(* Logix 5000 AddOnInstructionDefinition export YAI_Assy_155_119_EIP_Hz; software revision 21.03 *)

ADD_ON_INSTRUCTION YAI_Assy_155_119_EIP_Hz   (* revision 1.0, vendor Yaskawa America, Inc. *)
// YAI Assembly 155 and 119
// Help:
// This add-on instruction is for use with input assemblie 166 and output assemblies 116.
// Node_Input_Assy is defined as the node's input assembly integer array.
// Node_Output_Assy is defined as the node's output assembly integer array.
// Torque limit/reference, torque compensation and torque output variables are only available with A1000.
VAR_IN_OUT
   Node_Input_Assy : AB:ETHERNET_MODULE_INT_40Bytes:I:0; {required}   // Input assembly words
   Node_Output_Assy : AB:ETHERNET_MODULE_INT_18Bytes:O:0; {required}   // Output assembly words
END_VAR
VAR_INPUT
   RunFwd : BOOL; {visible}   // Forward run command
   RunRev : BOOL; {visible}   // Reverse run command
   MFI_3 : BOOL; {visible}   // Multi-function input 3
   MFI_4 : BOOL; {visible}   // Multi-function input 4
   MFI_5 : BOOL; {visible}   // Multi-function input 5
   MFI_6 : BOOL; {visible}   // Multi-function input 6
   MFI_7 : BOOL; {visible}   // Multi-function input 7
   MFI_8 : BOOL; {visible}   // Multi-function input 8
   External_Fault : BOOL;   // External fault command (EF0)
   FaultReset : BOOL; {visible}   // Fault reset command
   MFO_1 : BOOL; {visible}   // Multi-function output (M1-M2 for A/P1000, MA/MB/MC for V1000)
   MFO_2 : BOOL; {visible}   // Multi-function output (M3-M4 for A/P1000, P1 for V1000)
   MFO_3 : BOOL; {visible}   // Multi-function output (M5-M6 for A/P1000, P2 for V1000)
   Freq_Ref : REAL; {visible}   // Frequency reference command in Hz (xx.xx resolution)
   Digital_Output_Fault_Enable : BOOL;   // Bit to enable control of fault output relay over the network
END_VAR
VAR_OUTPUT
   Running : BOOL; {access Read Only, visible}   // Drive running forward status bit
   ZSP : BOOL; {access Read Only, visible}   // Drive zero speed status bit
   RunningRev : BOOL; {access Read Only, visible}   // Drive running reverse status bit
   Reset : BOOL; {access Read Only, visible}   // Drive reset command status bit
   At_Speed : BOOL; {access Read Only, visible}   // Drive at commanded speed status bit
   Ready : BOOL; {access Read Only, visible}   // Drive ready status bit
   Alarm : BOOL; {access Read Only, visible}   // Drive alarm status bit
   Faulted : BOOL; {access Read Only, visible}   // Drive faulted status bit
   OPE : BOOL; {access Read Only}   // OPE alarm/fault present
   UV : BOOL; {access Read Only}   // Drive in UV (undervoltage) state status bit
   NetCtrlStatus : BOOL; {access Read Only, visible}   // Drive network run source status bit (1 = source coming from network)
   MFO_1_Status : BOOL; {access Read Only, visible}   // Drive multi-function output 1 (M1-M2 for A/P1000, MA/MB/MC for V1000) status
   MFO_2_Status : BOOL; {access Read Only, visible}   // Drive multi-function output 1 (M3-M4 for A/P1000, P1 for V1000) status
   MFO_3_Status : BOOL; {access Read Only, visible}   // Drive multi-function output 1 (M5-M6 for A/P1000, P2 for V1000) status
   ZSV : BOOL; {access Read Only, visible}   // Drive zero servo completed status bit
   Motor_Speed : REAL; {access Read Only, visible}   // Motor speed in Hz (xx.xx resolution)
   Torque_Actual : REAL; {access Read Only, visible}   // Drive torque output in % (xxx.x resolution)
   PG1_Count : INT; {access Read Only}   // Encoder feedback count
   Freq_Cmd : REAL; {access Read Only, visible}   // Commanded frequency in Hz (xx.xx resolution)
   Output_Freq : REAL; {access Read Only, visible}   // Drive output frequency in Hz (xx.xx resolution)
   Output_Current : REAL; {access Read Only, visible}   // Drive output current in A (xxx.x resolution)
   Analog_Input_1_Level : REAL; {access Read Only}   // Analog input 1 level in % (xxx.x resolution)
   DC_Bus_Volt : INT; {access Read Only, visible}   // DC bus voltage in Vdc (xxx resolution)
   Analog_Input_3_Level : REAL; {access Read Only}   // Analog input 3 level in % (xxx.x resolution)
   Analog_Input_2_Level : REAL; {access Read Only}   // Analog input 2 level in % (xxx.x resolution)
   S1_Status : BOOL; {access Read Only}   // Digital input S1 status
   S2_Status : BOOL; {access Read Only}   // Digital input S2 status
   S3_Status : BOOL; {access Read Only}   // Digital input S3 status
   S4_Status : BOOL; {access Read Only}   // Digital input S4 status
   S5_Status : BOOL; {access Read Only}   // Digital input S5 status
   S6_Status : BOOL; {access Read Only}   // Digital input S6 status
   S7_Status : BOOL; {access Read Only}   // Digital input S7 status
   S8_Status : BOOL; {access Read Only}   // Digital input S8 status
   PG2_Count : INT;   // Encoder 2 feedback count
   UV_Alarm : BOOL; {access Read Only}   // Undervoltage alarm
   OV_Alarm : BOOL; {access Read Only}   // Overvoltage alarm
   OH_Alarm : BOOL; {access Read Only}   // Overheat alarm
   OH2_Alarm : BOOL; {access Read Only}   // Drive overheat alarm
   OL3_Alarm : BOOL; {access Read Only}   // Overtorque detection 1 alarm
   OL4_Alarm : BOOL; {access Read Only}   // Overtorque detection 2 alarm
   EF_Alarm : BOOL; {access Read Only}   // Run command error alarm
   bb_Alarm : BOOL; {access Read Only}   // Baseblock alarm
   EF3_Alarm : BOOL; {access Read Only}   // External fault 3 alarm
   EF4_Alarm : BOOL; {access Read Only}   // External fault 4 alarm
   EF5_Alarm : BOOL; {access Read Only}   // External fault 5 alarm
   EF6_Alarm : BOOL; {access Read Only}   // External fault 6 alarm
   EF7_Alarm : BOOL; {access Read Only}   // External fault 7 alarm
   EF8_Alarm : BOOL; {access Read Only}   // External fault 8 alarm
   FAN_Alarm : BOOL; {access Read Only}   // Cooling fan error alarm
   OS_Alarm : BOOL; {access Read Only}   // Overspeed alarm
   DEV_Alarm : BOOL; {access Read Only}   // Speed deviation alarm
   PGO_Alarm : BOOL; {access Read Only}   // Encoder feedback open alarm
   OPR_Alarm : BOOL; {access Read Only}   // Operator removed alarm
   CE_Alarm : BOOL; {access Read Only}   // Serial communication error alarm
   BUS_Alarm : BOOL; {access Read Only}   // BUS alarm
   CALL_Alarm : BOOL; {access Read Only}   // Serial communication timeout alarm
   OL1_Alarm : BOOL; {access Read Only}   // Motor overload alarm
   OL2_Alarm : BOOL; {access Read Only}   // Drive overload alarm
   EF0_Alarm : BOOL; {access Read Only}   // External fault 0 alarm
   RUN_Alarm : BOOL; {access Read Only}   // Motor 2 run command issued while running alarm
   UL3_Alarm : BOOL; {access Read Only}   // Undertorque detecxtion 1 alarm
   UL4_Alarm : BOOL; {access Read Only}   // Undertorque detection 2 alarm
   SE_Alarm : BOOL; {access Read Only}   // Modbus test failure alarm
   OH3_Alarm : BOOL; {access Read Only}   // Motor overload alarm
   FBL_Alarm : BOOL; {access Read Only}   // PID feedback loss alarm
   FBH_Alarm : BOOL; {access Read Only}   // PID feedback loss alarm
   DNE_Alarm : BOOL; {access Read Only}   // Drive not enabled alarm
END_VAR
VAR_INPUT
   Custom_Out_1 : INT;
   Custom_Out_2 : INT;
   Custom_Out_3 : INT;
   Custom_Out_4 : INT;
   Custom_Out_5 : INT;
   Custom_Out_6 : INT;
   Custom_Out_7 : INT;
END_VAR
VAR
   FRef_Convert : DINT;
   FOut_Convert : REAL;
   FOut_Temp : REAL;
   TRef_Convert : INT;
   TComp_Convert : INT;
   TOut_Convert : REAL;
   TOut_Temp : REAL;
   IOut_Temp : REAL;
   IOut_Convert : REAL;
   AO1_Convert : INT;
   AO2_Convert : INT;
   Motor_Speed_Temp : REAL;
   Motor_Speed_Convert : REAL;
   Freq_Cmd_Temp : REAL;
   Freq_Cmd_Convert : REAL;
   AI1_Temp : REAL;
   AI1_Convert : REAL;
   AI2_Temp : REAL; {access None}
   AI2_Convert : REAL; {access None}
   AI3_Temp : REAL; {access None}
   AI3_Convert : REAL; {access None}
END_VAR

ROUTINE Logic   (* ladder *)
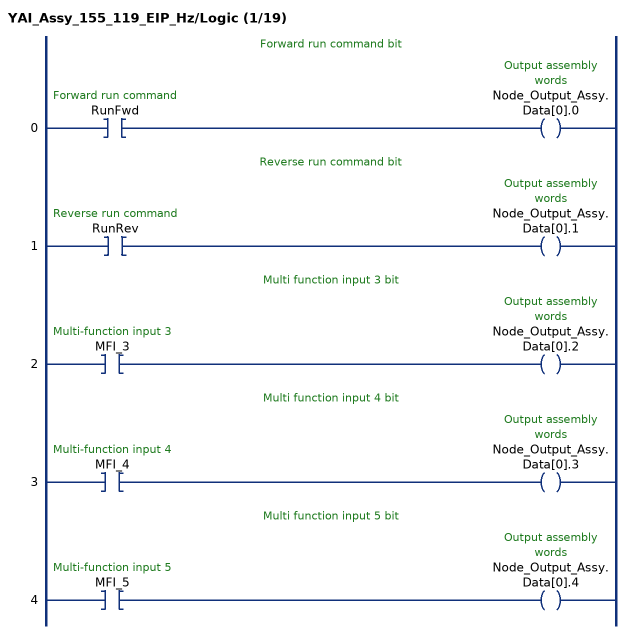
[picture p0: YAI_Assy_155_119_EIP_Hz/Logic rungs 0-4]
   // Forward run command bit
   0: XIC(RunFwd)OTE(Node_Output_Assy.Data[0].0);
   // Reverse run command bit
   1: XIC(RunRev)OTE(Node_Output_Assy.Data[0].1);
   // Multi function input 3 bit
   2: XIC(MFI_3)OTE(Node_Output_Assy.Data[0].2);
   // Multi function input 4 bit
   3: XIC(MFI_4)OTE(Node_Output_Assy.Data[0].3);
   // Multi function input 5 bit
   4: XIC(MFI_5)OTE(Node_Output_Assy.Data[0].4);
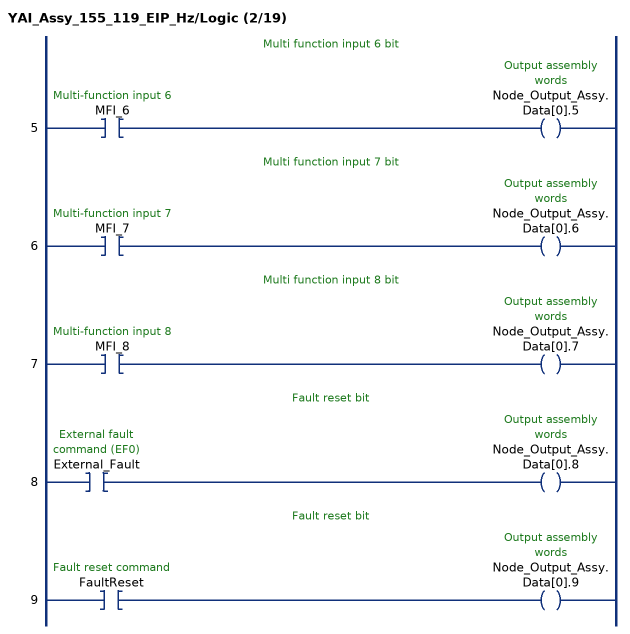
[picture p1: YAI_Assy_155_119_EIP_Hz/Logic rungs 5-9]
   // Multi function input 6 bit
   5: XIC(MFI_6)OTE(Node_Output_Assy.Data[0].5);
   // Multi function input 7 bit
   6: XIC(MFI_7)OTE(Node_Output_Assy.Data[0].6);
   // Multi function input 8 bit
   7: XIC(MFI_8)OTE(Node_Output_Assy.Data[0].7);
   // Fault reset bit
   8: XIC(External_Fault)OTE(Node_Output_Assy.Data[0].8);
   // Fault reset bit
   9: XIC(FaultReset)OTE(Node_Output_Assy.Data[0].9);
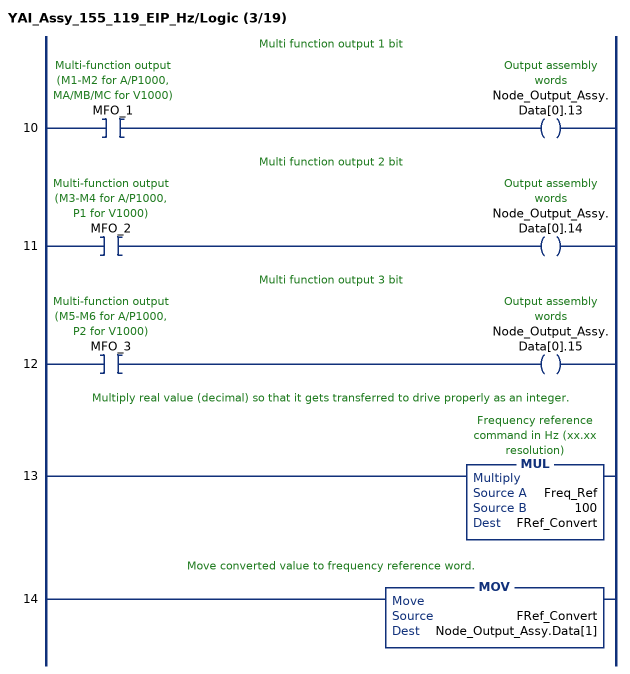
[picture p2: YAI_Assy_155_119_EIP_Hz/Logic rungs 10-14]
   // Multi function output 1 bit
   10: XIC(MFO_1)OTE(Node_Output_Assy.Data[0].13);
   // Multi function output 2 bit
   11: XIC(MFO_2)OTE(Node_Output_Assy.Data[0].14);
   // Multi function output 3 bit
   12: XIC(MFO_3)OTE(Node_Output_Assy.Data[0].15);
   // Multiply real value (decimal) so that it gets transferred to drive properly as an integer.
   13: MUL(Freq_Ref,100,FRef_Convert);
   // Move converted value to frequency reference word.
   14: MOV(FRef_Convert,Node_Output_Assy.Data[1]);
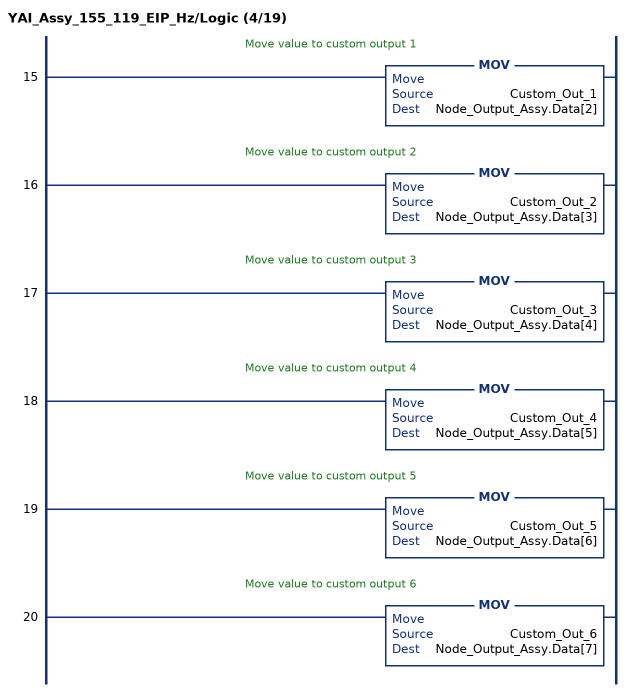
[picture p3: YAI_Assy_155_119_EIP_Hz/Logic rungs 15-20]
   // Move value to custom output 1
   15: MOV(Custom_Out_1,Node_Output_Assy.Data[2]);
   // Move value to custom output 2
   16: MOV(Custom_Out_2,Node_Output_Assy.Data[3]);
   // Move value to custom output 3
   17: MOV(Custom_Out_3,Node_Output_Assy.Data[4]);
   // Move value to custom output 4
   18: MOV(Custom_Out_4,Node_Output_Assy.Data[5]);
   // Move value to custom output 5
   19: MOV(Custom_Out_5,Node_Output_Assy.Data[6]);
   // Move value to custom output 6
   20: MOV(Custom_Out_6,Node_Output_Assy.Data[7]);
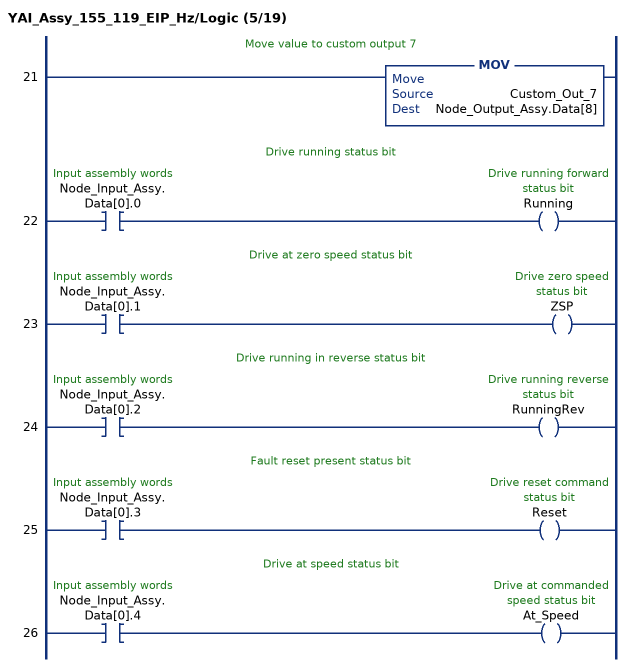
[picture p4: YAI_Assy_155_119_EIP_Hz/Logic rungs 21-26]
   // Move value to custom output 7
   21: MOV(Custom_Out_7,Node_Output_Assy.Data[8]);
   // Drive running status bit
   22: XIC(Node_Input_Assy.Data[0].0)OTE(Running);
   // Drive at zero speed status bit
   23: XIC(Node_Input_Assy.Data[0].1)OTE(ZSP);
   // Drive running in reverse status bit
   24: XIC(Node_Input_Assy.Data[0].2)OTE(RunningRev);
   // Fault reset present status bit
   25: XIC(Node_Input_Assy.Data[0].3)OTE(Reset);
   // Drive at speed status bit
   26: XIC(Node_Input_Assy.Data[0].4)OTE(At_Speed);
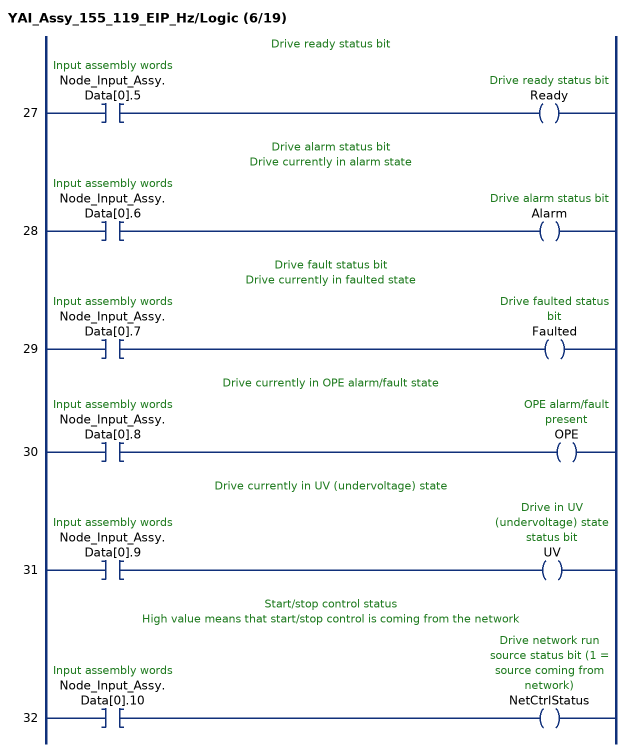
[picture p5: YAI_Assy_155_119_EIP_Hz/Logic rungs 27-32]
   // Drive ready status bit
   27: XIC(Node_Input_Assy.Data[0].5)OTE(Ready);
   // Drive alarm status bit
   // Drive currently in alarm state
   28: XIC(Node_Input_Assy.Data[0].6)OTE(Alarm);
   // Drive fault status bit
   // Drive currently in faulted state
   29: XIC(Node_Input_Assy.Data[0].7)OTE(Faulted);
   // Drive currently in OPE alarm/fault state
   30: XIC(Node_Input_Assy.Data[0].8)OTE(OPE);
   // Drive currently in UV (undervoltage) state
   31: XIC(Node_Input_Assy.Data[0].9)OTE(UV);
   // Start/stop control status
   // High value means that start/stop control is coming from the network
   32: XIC(Node_Input_Assy.Data[0].10)OTE(NetCtrlStatus);
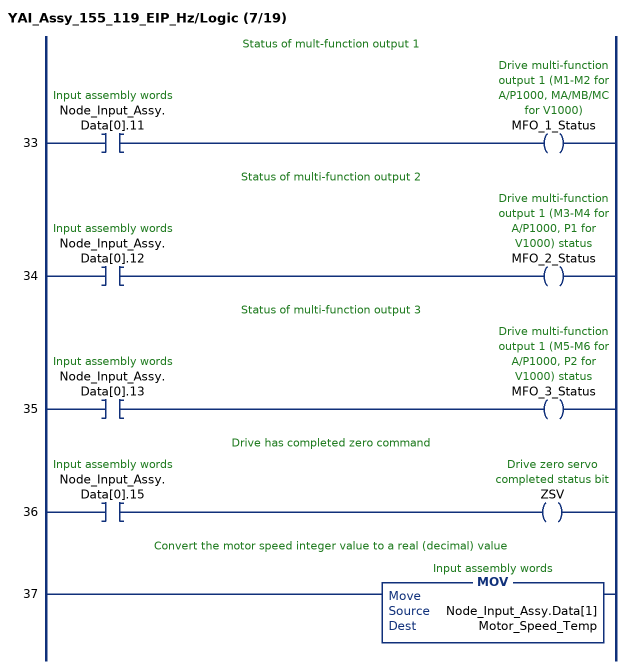
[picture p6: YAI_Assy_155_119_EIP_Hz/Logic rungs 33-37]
   // Status of mult-function output 1
   33: XIC(Node_Input_Assy.Data[0].11)OTE(MFO_1_Status);
   // Status of multi-function output 2
   34: XIC(Node_Input_Assy.Data[0].12)OTE(MFO_2_Status);
   // Status of multi-function output 3
   35: XIC(Node_Input_Assy.Data[0].13)OTE(MFO_3_Status);
   // Drive has completed zero command
   36: XIC(Node_Input_Assy.Data[0].15)OTE(ZSV);
   // Convert the motor speed integer value to a real (decimal) value
   37: MOV(Node_Input_Assy.Data[1],Motor_Speed_Temp);
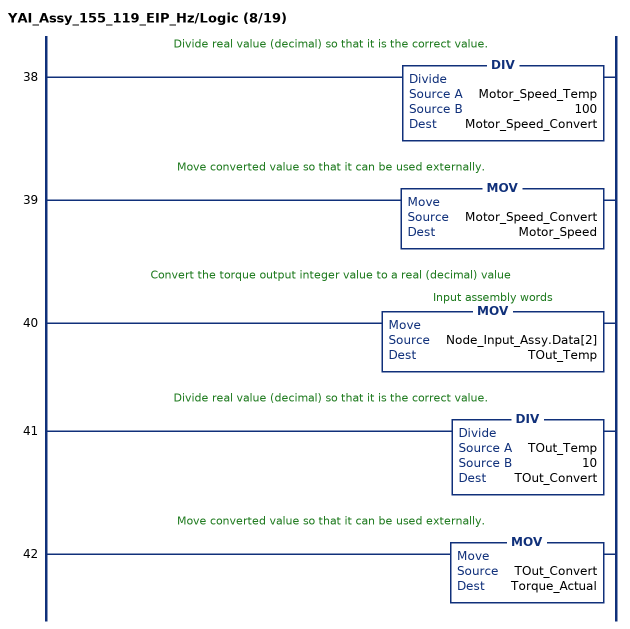
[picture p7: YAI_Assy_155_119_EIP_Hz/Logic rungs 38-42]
   // Divide real value (decimal) so that it is the correct value.
   38: DIV(Motor_Speed_Temp,100,Motor_Speed_Convert);
   // Move converted value so that it can be used externally.
   39: MOV(Motor_Speed_Convert,Motor_Speed);
   // Convert the torque output integer value to a real (decimal) value
   40: MOV(Node_Input_Assy.Data[2],TOut_Temp);
   // Divide real value (decimal) so that it is the correct value.
   41: DIV(TOut_Temp,10,TOut_Convert);
   // Move converted value so that it can be used externally.
   42: MOV(TOut_Convert,Torque_Actual);
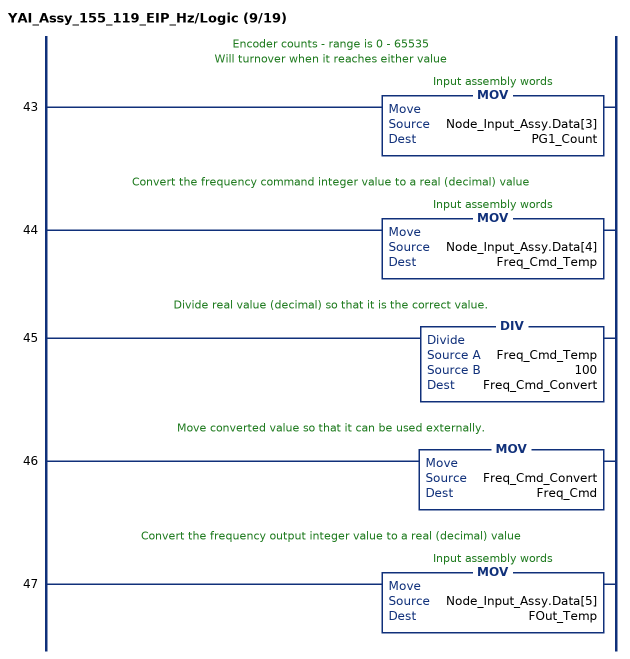
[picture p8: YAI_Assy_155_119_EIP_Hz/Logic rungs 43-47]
   // Encoder counts - range is 0 - 65535
   // Will turnover when it reaches either value
   43: MOV(Node_Input_Assy.Data[3],PG1_Count);
   // Convert the frequency command integer value to a real (decimal) value
   44: MOV(Node_Input_Assy.Data[4],Freq_Cmd_Temp);
   // Divide real value (decimal) so that it is the correct value.
   45: DIV(Freq_Cmd_Temp,100,Freq_Cmd_Convert);
   // Move converted value so that it can be used externally.
   46: MOV(Freq_Cmd_Convert,Freq_Cmd);
   // Convert the frequency output integer value to a real (decimal) value
   47: MOV(Node_Input_Assy.Data[5],FOut_Temp);
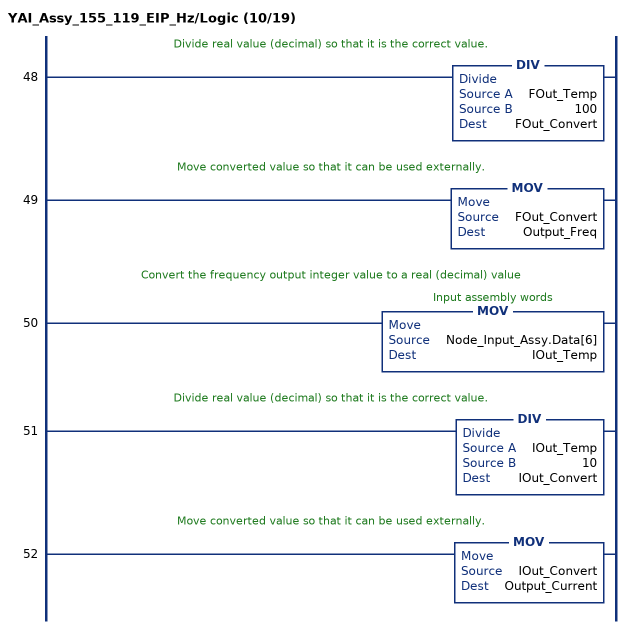
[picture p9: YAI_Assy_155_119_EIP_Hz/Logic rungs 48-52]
   // Divide real value (decimal) so that it is the correct value.
   48: DIV(FOut_Temp,100,FOut_Convert);
   // Move converted value so that it can be used externally.
   49: MOV(FOut_Convert,Output_Freq);
   // Convert the frequency output integer value to a real (decimal) value
   50: MOV(Node_Input_Assy.Data[6],IOut_Temp);
   // Divide real value (decimal) so that it is the correct value.
   51: DIV(IOut_Temp,10,IOut_Convert);
   // Move converted value so that it can be used externally.
   52: MOV(IOut_Convert,Output_Current);
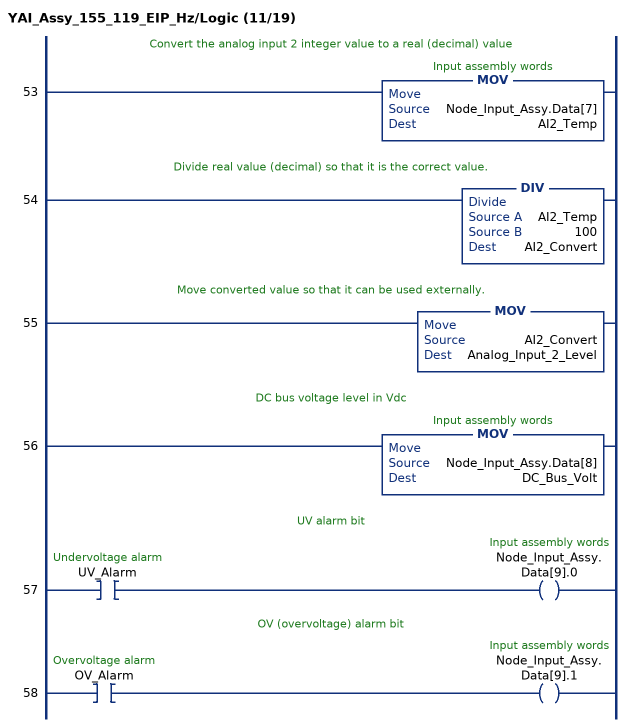
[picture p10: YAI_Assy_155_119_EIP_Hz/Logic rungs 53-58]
   // Convert the analog input 2 integer value to a real (decimal) value
   53: MOV(Node_Input_Assy.Data[7],AI2_Temp);
   // Divide real value (decimal) so that it is the correct value.
   54: DIV(AI2_Temp,100,AI2_Convert);
   // Move converted value so that it can be used externally.
   55: MOV(AI2_Convert,Analog_Input_2_Level);
   // DC bus voltage level in Vdc
   56: MOV(Node_Input_Assy.Data[8],DC_Bus_Volt);
   // UV alarm bit
   57: XIC(UV_Alarm)OTE(Node_Input_Assy.Data[9].0);
   // OV (overvoltage) alarm bit
   58: XIC(OV_Alarm)OTE(Node_Input_Assy.Data[9].1);
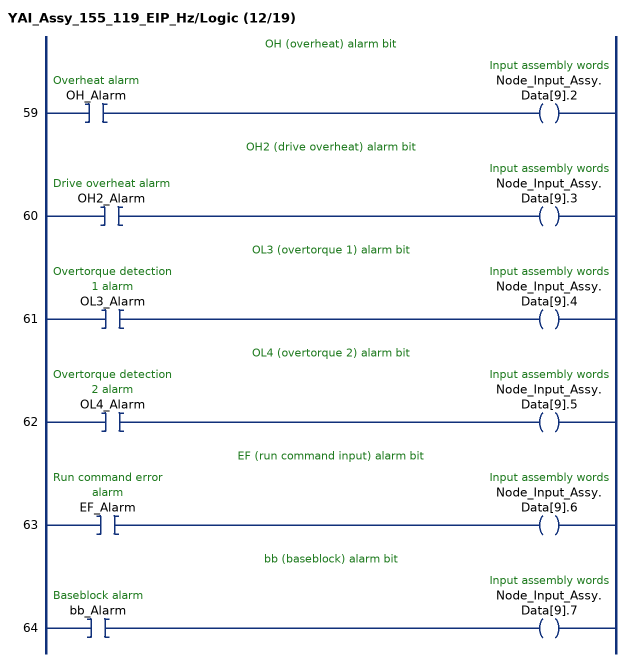
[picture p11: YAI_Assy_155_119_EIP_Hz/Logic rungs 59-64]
   // OH (overheat) alarm bit
   59: XIC(OH_Alarm)OTE(Node_Input_Assy.Data[9].2);
   // OH2 (drive overheat) alarm bit
   60: XIC(OH2_Alarm)OTE(Node_Input_Assy.Data[9].3);
   // OL3 (overtorque 1) alarm bit
   61: XIC(OL3_Alarm)OTE(Node_Input_Assy.Data[9].4);
   // OL4 (overtorque 2) alarm bit
   62: XIC(OL4_Alarm)OTE(Node_Input_Assy.Data[9].5);
   // EF (run command input) alarm bit
   63: XIC(EF_Alarm)OTE(Node_Input_Assy.Data[9].6);
   // bb (baseblock) alarm bit
   64: XIC(bb_Alarm)OTE(Node_Input_Assy.Data[9].7);
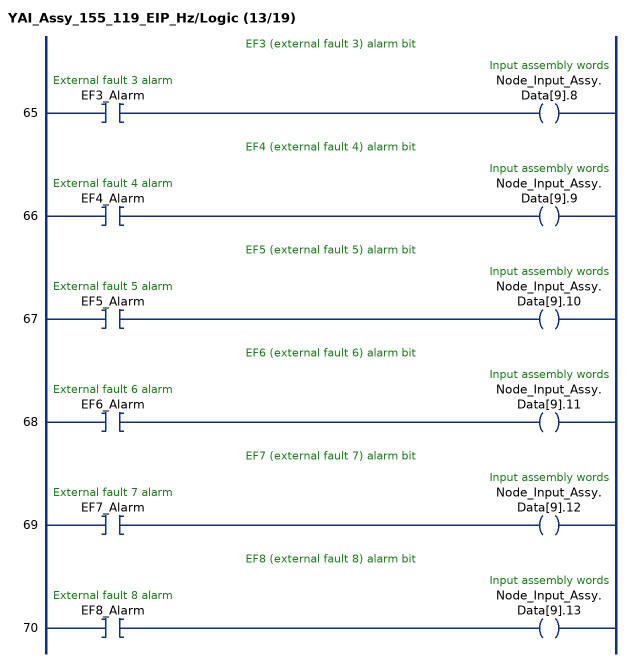
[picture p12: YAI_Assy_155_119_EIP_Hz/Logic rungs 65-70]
   // EF3 (external fault 3) alarm bit
   65: XIC(EF3_Alarm)OTE(Node_Input_Assy.Data[9].8);
   // EF4 (external fault 4) alarm bit
   66: XIC(EF4_Alarm)OTE(Node_Input_Assy.Data[9].9);
   // EF5 (external fault 5) alarm bit
   67: XIC(EF5_Alarm)OTE(Node_Input_Assy.Data[9].10);
   // EF6 (external fault 6) alarm bit
   68: XIC(EF6_Alarm)OTE(Node_Input_Assy.Data[9].11);
   // EF7 (external fault 7) alarm bit
   69: XIC(EF7_Alarm)OTE(Node_Input_Assy.Data[9].12);
   // EF8 (external fault 8) alarm bit
   70: XIC(EF8_Alarm)OTE(Node_Input_Assy.Data[9].13);
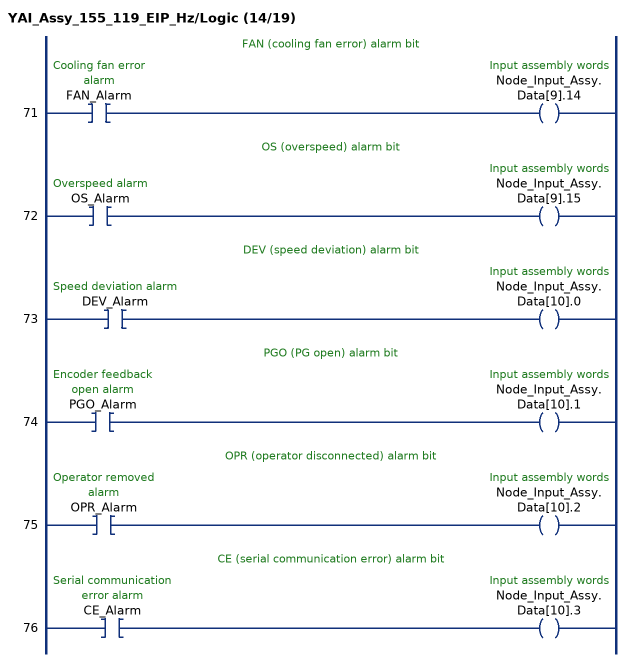
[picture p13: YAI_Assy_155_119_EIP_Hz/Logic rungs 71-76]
   // FAN (cooling fan error) alarm bit
   71: XIC(FAN_Alarm)OTE(Node_Input_Assy.Data[9].14);
   // OS (overspeed) alarm bit
   72: XIC(OS_Alarm)OTE(Node_Input_Assy.Data[9].15);
   // DEV (speed deviation) alarm bit
   73: XIC(DEV_Alarm)OTE(Node_Input_Assy.Data[10].0);
   // PGO (PG open) alarm bit
   74: XIC(PGO_Alarm)OTE(Node_Input_Assy.Data[10].1);
   // OPR (operator disconnected) alarm bit
   75: XIC(OPR_Alarm)OTE(Node_Input_Assy.Data[10].2);
   // CE (serial communication error) alarm bit
   76: XIC(CE_Alarm)OTE(Node_Input_Assy.Data[10].3);
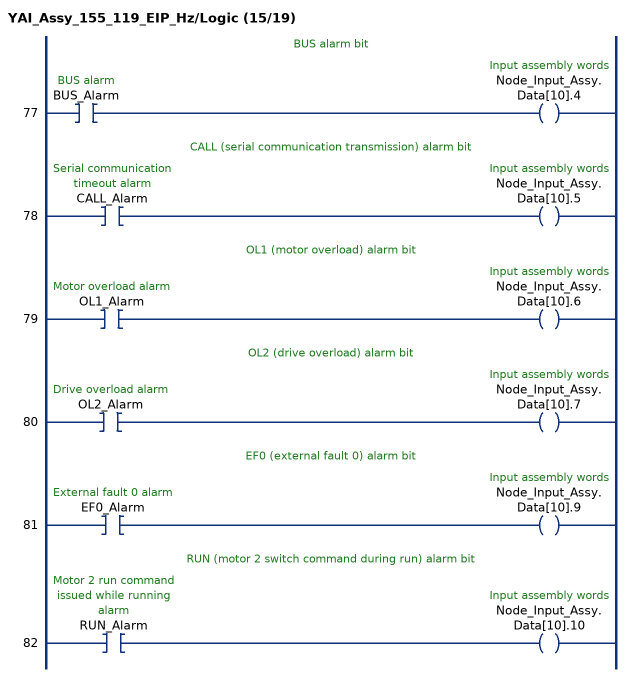
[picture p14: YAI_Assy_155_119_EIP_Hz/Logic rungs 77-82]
   // BUS alarm bit
   77: XIC(BUS_Alarm)OTE(Node_Input_Assy.Data[10].4);
   // CALL (serial communication transmission) alarm bit
   78: XIC(CALL_Alarm)OTE(Node_Input_Assy.Data[10].5);
   // OL1 (motor overload) alarm bit
   79: XIC(OL1_Alarm)OTE(Node_Input_Assy.Data[10].6);
   // OL2 (drive overload) alarm bit
   80: XIC(OL2_Alarm)OTE(Node_Input_Assy.Data[10].7);
   // EF0 (external fault 0) alarm bit
   81: XIC(EF0_Alarm)OTE(Node_Input_Assy.Data[10].9);
   // RUN (motor 2 switch command during run) alarm bit
   82: XIC(RUN_Alarm)OTE(Node_Input_Assy.Data[10].10);
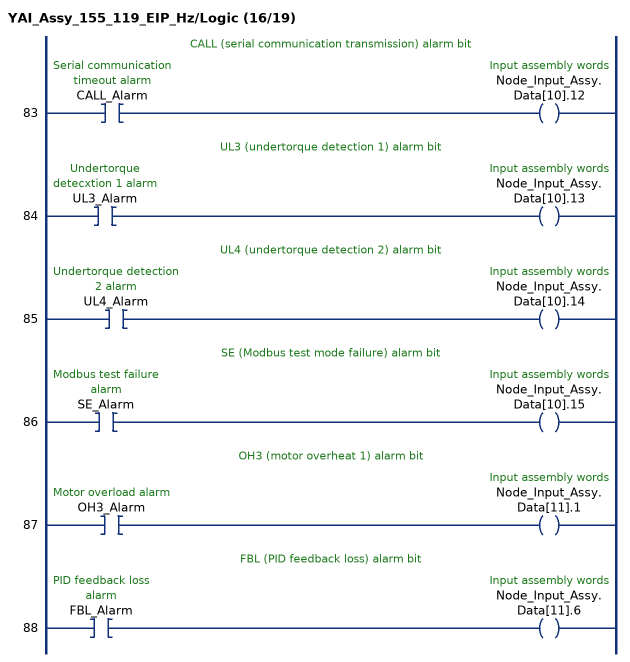
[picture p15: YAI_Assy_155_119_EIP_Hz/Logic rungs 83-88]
   // CALL (serial communication transmission) alarm bit
   83: XIC(CALL_Alarm)OTE(Node_Input_Assy.Data[10].12);
   // UL3 (undertorque detection 1) alarm bit
   84: XIC(UL3_Alarm)OTE(Node_Input_Assy.Data[10].13);
   // UL4 (undertorque detection 2) alarm bit
   85: XIC(UL4_Alarm)OTE(Node_Input_Assy.Data[10].14);
   // SE (Modbus test mode failure) alarm bit
   86: XIC(SE_Alarm)OTE(Node_Input_Assy.Data[10].15);
   // OH3 (motor overheat 1) alarm bit
   87: XIC(OH3_Alarm)OTE(Node_Input_Assy.Data[11].1);
   // FBL (PID feedback loss) alarm bit
   88: XIC(FBL_Alarm)OTE(Node_Input_Assy.Data[11].6);
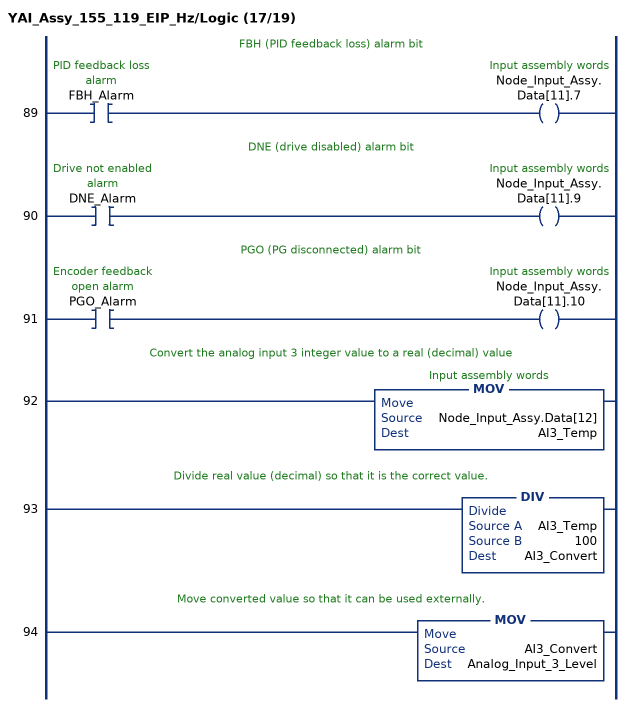
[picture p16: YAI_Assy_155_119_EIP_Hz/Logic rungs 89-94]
   // FBH (PID feedback loss) alarm bit
   89: XIC(FBH_Alarm)OTE(Node_Input_Assy.Data[11].7);
   // DNE (drive disabled) alarm bit
   90: XIC(DNE_Alarm)OTE(Node_Input_Assy.Data[11].9);
   // PGO (PG disconnected) alarm bit
   91: XIC(PGO_Alarm)OTE(Node_Input_Assy.Data[11].10);
   // Convert the analog input 3 integer value to a real (decimal) value
   92: MOV(Node_Input_Assy.Data[12],AI3_Temp);
   // Divide real value (decimal) so that it is the correct value.
   93: DIV(AI3_Temp,100,AI3_Convert);
   // Move converted value so that it can be used externally.
   94: MOV(AI3_Convert,Analog_Input_3_Level);
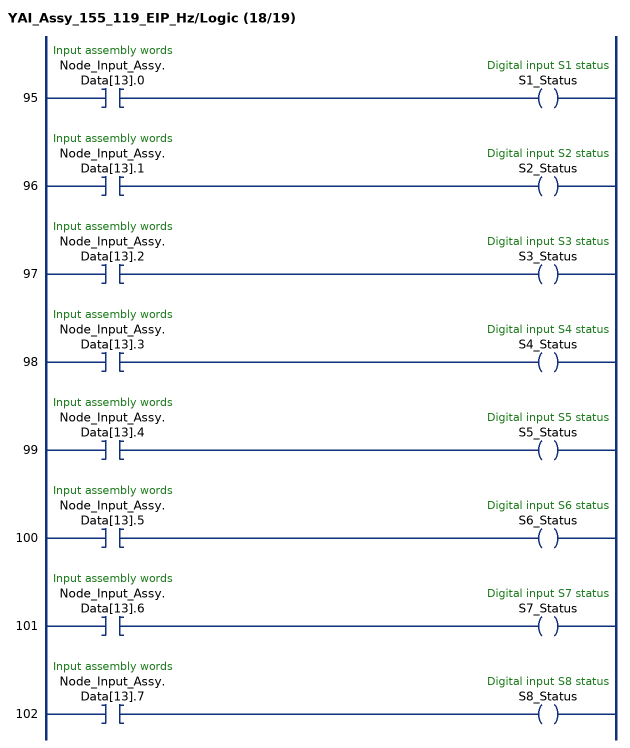
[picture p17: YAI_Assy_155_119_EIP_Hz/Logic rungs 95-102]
   95: XIC(Node_Input_Assy.Data[13].0)OTE(S1_Status);
   96: XIC(Node_Input_Assy.Data[13].1)OTE(S2_Status);
   97: XIC(Node_Input_Assy.Data[13].2)OTE(S3_Status);
   98: XIC(Node_Input_Assy.Data[13].3)OTE(S4_Status);
   99: XIC(Node_Input_Assy.Data[13].4)OTE(S5_Status);
   100: XIC(Node_Input_Assy.Data[13].5)OTE(S6_Status);
   101: XIC(Node_Input_Assy.Data[13].6)OTE(S7_Status);
   102: XIC(Node_Input_Assy.Data[13].7)OTE(S8_Status);
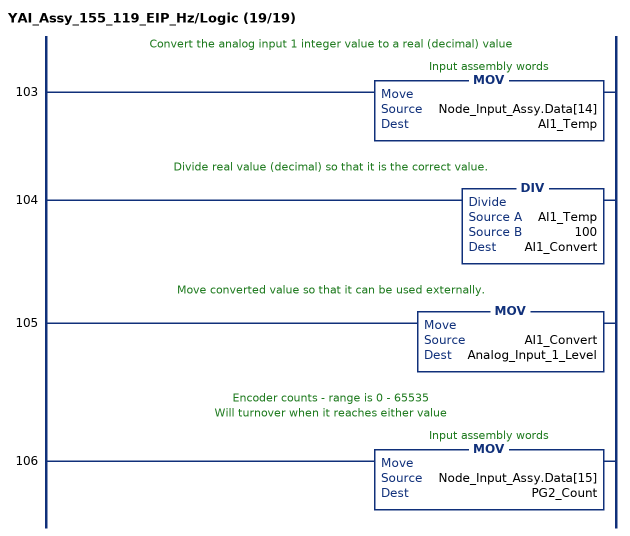
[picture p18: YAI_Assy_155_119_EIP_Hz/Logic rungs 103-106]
   // Convert the analog input 1 integer value to a real (decimal) value
   103: MOV(Node_Input_Assy.Data[14],AI1_Temp);
   // Divide real value (decimal) so that it is the correct value.
   104: DIV(AI1_Temp,100,AI1_Convert);
   // Move converted value so that it can be used externally.
   105: MOV(AI1_Convert,Analog_Input_1_Level);
   // Encoder counts - range is 0 - 65535
   // Will turnover when it reaches either value
   106: MOV(Node_Input_Assy.Data[15],PG2_Count);
END_ROUTINE
END_ADD_ON_INSTRUCTION
